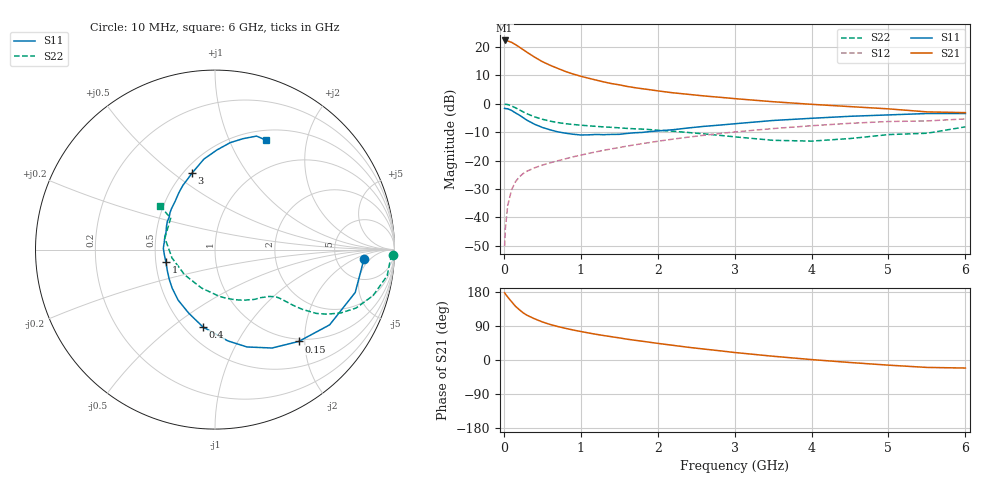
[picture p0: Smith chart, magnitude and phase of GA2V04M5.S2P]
! Infineon Technologies  Discrete & RF Semiconductors
! BF775
! Si NPN RF Bipolar Junction Transistor in SOT23
! VCE = 2 V  IC = 4.5 mA
! Common Emitter S-Parameters:  May  1996
# GHz  S  MA  R  50
!  f  S11  S21  S12  S22
! GHz  MAG  ANG  MAG  ANG  MAG  ANG  MAG  ANG
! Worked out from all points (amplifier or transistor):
!   36 points, 10 MHz to 6 GHz, reference 50 ohm
!   highest |S21| = 22.3 dB at 10 MHz (marker M1)
!   |S21| within 3 dB of that: start of sweep to 237.7 MHz
!   unconditionally stable (mu >= 1): 791 MHz to 4.038 GHz; 5.338 GHz to 5.791 GHz
!   at 250 MHz: K = 0.47, MSG = 21.9 dB, |S12| = -24.6 dB
!   at 1.4 GHz: K = 1.14, MAG = 9.2 dB, |S12| = -15.9 dB
!   at 6 GHz: K = 0.99, MSG = 1.1 dB, |S12| = -5.3 dB
!   S11 on the Smith chart (normalised r, x): 10 MHz: 10, -3; 150 MHz: 0.95, -1.87; 400 MHz: 0.61, -0.65; 1 GHz: 0.57, -0.08; 3 GHz: 0.55, +0.59; 6 GHz: 0.62, +1.38
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0.01  0.8309 -3.5  13.06 177.4  0.0031 87.0  0.9908 -1.7
0.02  0.8235 -7.1  13.04 174.3  0.0064 86.4  0.9782 -3.5
0.05  0.817 -17.0  12.8 166.3  0.0161 80.4  0.9704 -8.6
0.1  0.7639 -33.3  12.11 153.9  0.0304 72.7  0.9174 -16.2
0.15  0.6926 -47.6  11.06 142.0  0.0421 65.8  0.8507 -22.5
0.2  0.6338 -59.9  10 133.0  0.0514 62.0  0.7853 -26.7
0.25  0.571 -71.8  9.009 124.7  0.0588 57.9  0.7219 -29.9
0.3  0.5141 -81.9  8.102 118.2  0.0648 56.0  0.6674 -32.2
0.4  0.4359 -98.9  6.627 108.7  0.0745 53.6  0.5886 -34.4
0.5  0.3834 -112.4  5.532 100.5  0.0831 52.8  0.5338 -35.5
0.6  0.3483 -126.2  4.787 93.9  0.091 52.6  0.4953 -36.1
0.8  0.3036 -147.2  3.716 83.6  0.1072 53.4  0.4465 -37.1
1  0.282 -166.1  3.057 75.2  0.1244 54.0  0.4203 -38.5
1.1  0.2837 -174.3  2.824 71.4  0.1336 54.2  0.4096 -39.7
1.3  0.2856 171.9  2.427 64.5  0.1518 54.1  0.3914 -41.9
1.6  0.3002 154.2  2.025 55.0  0.1795 53.4  0.3686 -46.6
2.2  0.3493 129.4  1.56 38.7  0.2386 49.7  0.3283 -59.0
3  0.4446 106.8  1.233 19.8  0.319 41.6  0.2616 -84.7
3.5  0.508 97.0  1.087 9.9  0.3659 35.5  0.2272 -109.0
4.5  0.6019 81.9  0.892 -6.6  0.4528 22.5  0.2442 -169.1
5.5  0.6735 69.9  0.72 -19.6  0.4988 7.7  0.3026 144.7
6  0.6724 64.9  0.698 -21.2  0.5415 3.7  0.3926 141.4
